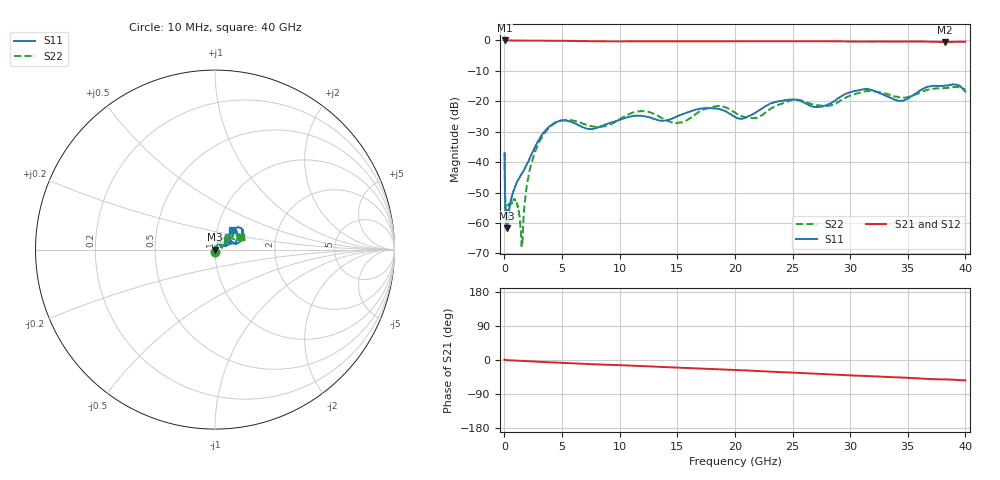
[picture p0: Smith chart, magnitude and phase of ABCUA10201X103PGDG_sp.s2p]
! Amotech Co.,Ltd.
! http://www.amotech.co.kr/
! Date: Wednesday, December 02, 2020 15:21:56
! Part Number: ABCUA 102 01X 103P GDG
! Freq. Start=10[MHz] Stop=40[GHz], 4000[Steps]
# Hz S  dB  R 50
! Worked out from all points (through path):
!   4000 points, 10 MHz to 40 GHz, reference 50 ohm
!   highest |S21| = -0.01 dB at 40 MHz (marker M1); lowest = -0.5 dB at 38.21 GHz (marker M2)
!   group delay of S21, straight-line fit = 3.69 ps
!   lowest |S11| = -61.7 dB at 200 MHz (marker M3), VSWR 1.00, Z = 50.1 - j0.0583 ohm
!   |S11| at or under -10 dB: start of sweep to end of sweep
!   |S22| runs from -67.6 to -15.2 dB; largest |S21 - S12| = 0.002
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1e7  -37.01 -88.8  -0.01 0.8  -0.00 0.8  -36.95 -83.6
4e7  -49.47 -85.8  -0.01 0.1  -0.00 0.1  -48.85 -70.4
2e8  -61.71 -45.1  -0.01 -0.3  -0.01 -0.3  -56.71 -21.9
3.2e8  -58.77 -32.0  -0.02 -0.6  -0.01 -0.5  -54.30 -19.8
9.8e8  -47.47 -19.6  -0.03 -1.6  -0.03 -1.6  -53.08 -43.9
1.5e9  -43.72 0.5  -0.04 -2.4  -0.04 -2.4  -67.12 17.0
2.16e9  -38.91 34.2  -0.05 -3.4  -0.04 -3.3  -43.06 98.3
3.18e9  -31.42 61.4  -0.07 -4.9  -0.06 -4.9  -32.30 86.5
4.72e9  -26.54 70.9  -0.11 -7.4  -0.11 -7.4  -26.51 69.7
6.68e9  -28.28 51.6  -0.23 -10.1  -0.22 -10.1  -27.18 39.7
1.167e10  -24.71 53.9  -0.30 -15.7  -0.29 -15.7  -23.25 35.5
1.334e10  -26.19 43.7  -0.30 -17.9  -0.29 -17.9  -24.79 34.0
1.522e10  -24.57 19.2  -0.32 -20.3  -0.31 -20.3  -27.04 40.2
1.744e10  -22.28 44.4  -0.32 -23.0  -0.31 -23.0  -22.49 38.9
2.001e10  -25.22 51.1  -0.27 -26.3  -0.26 -26.2  -23.72 33.4
2.181e10  -23.66 20.1  -0.25 -28.9  -0.24 -28.9  -25.41 55.0
2.451e10  -19.53 43.5  -0.27 -32.6  -0.27 -32.6  -20.12 42.2
2.667e10  -21.68 44.4  -0.26 -35.6  -0.25 -35.6  -20.92 36.0
3.12e10  -16.00 41.4  -0.39 -42.0  -0.38 -41.9  -16.81 31.9
3.334e10  -18.59 45.7  -0.37 -44.9  -0.36 -44.9  -17.78 24.2
3.821e10  -14.86 32.1  -0.50 -51.2  -0.49 -51.2  -15.63 22.0
4e10  -16.80 49.2  -0.41 -53.7  -0.40 -53.7  -15.99 26.8
